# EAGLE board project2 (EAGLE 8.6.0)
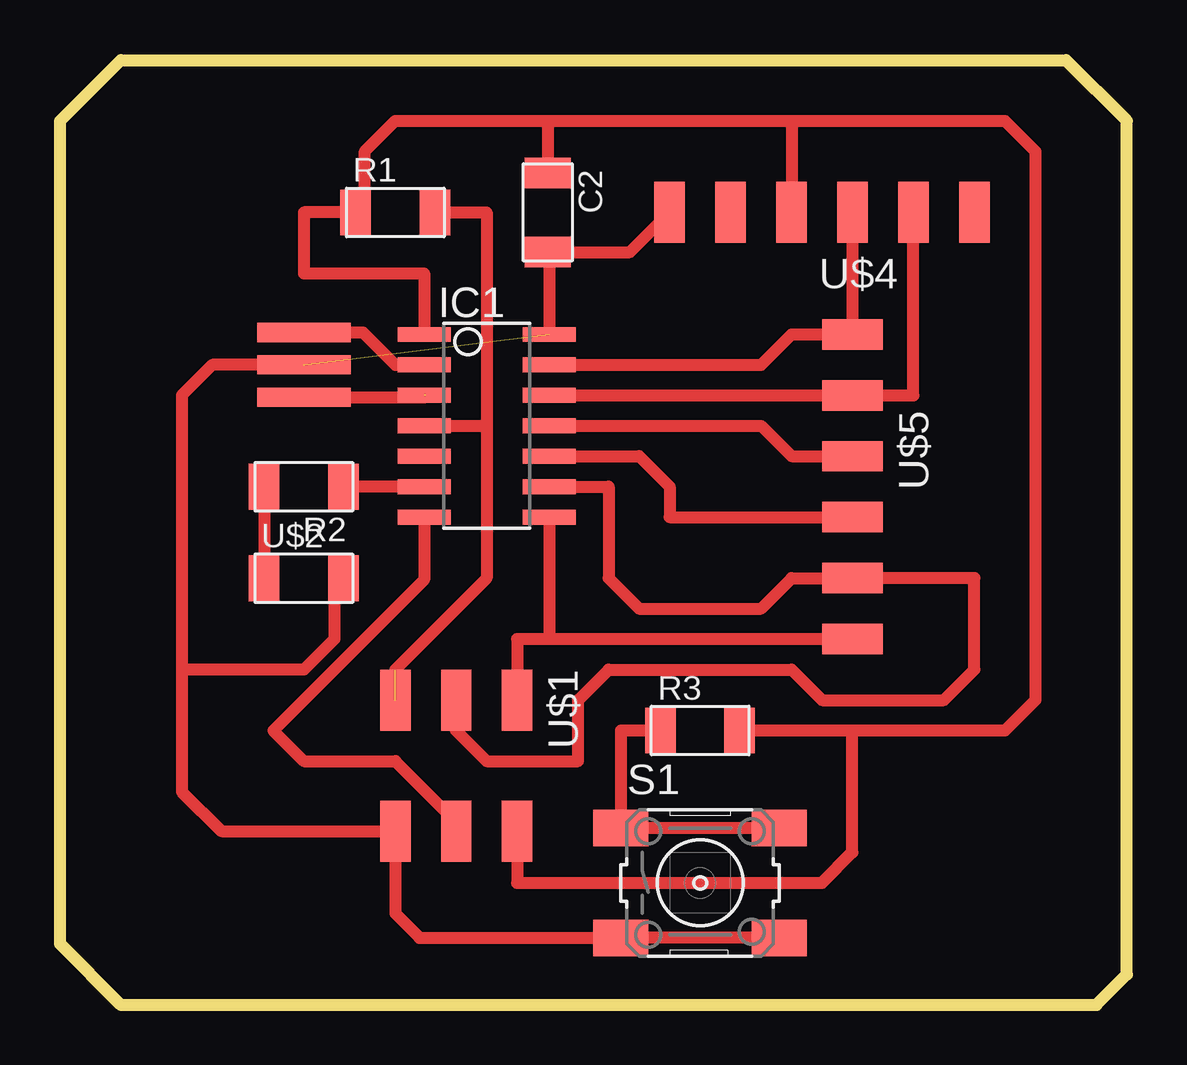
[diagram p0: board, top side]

Size 44.45 x 39.37 mm. Coordinates in mm from the lower left corner, seen from the top.
Outline: 2.54,0 43.18,0 44.45,1.27 44.45,36.83 41.91,39.37 2.54,39.37 0,36.83 0,2.54 2.54,0
Copper layers (1*16): Top 0.035mm / dielectric 1.5mm / Bottom 0.035mm
Design rules "default": minimum track width 6mil, minimum drill 0.35mm, track to track 6mil, track to pad 6mil, pad to pad 6mil, via to via 6mil, smd to smd 6mil, copper to edge 40mil, drill to drill 6mil, minimum pad ring 10mil, minimum via ring 8mil, stop-mask expansion 4mil, vias tented up to drill 0mil, thermal gap 10mil

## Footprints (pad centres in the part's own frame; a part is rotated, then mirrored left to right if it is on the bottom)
C1206FAB = smd 1.27 x 1.905: 1 -1.651,0; 2 1.651,0
SOIC14 = smd 0.61 x 2.21: 1 -3.81,-2.603; 2 -2.54,-2.603; 3 -1.27,-2.603; 4 0,-2.603; 5 1.27,-2.603; 6 2.54,-2.603; 7 3.81,-2.603; 8 3.81,2.603; 9 2.54,2.603; 10 1.27,2.603; 11 0,2.603; 12 -1.27,2.603; 13 -2.54,2.603; 14 -3.81,2.603
R1206FAB = smd 1.27 x 1.905: 1 -1.651,0; 2 1.651,0
6MM_SWITCH = smd 2.286 x 1.524: 1 -3.302,2.286; 2 3.302,2.286; 3 -3.302,-2.286; 4 3.302,-2.286
2X03SMD = smd 2.54 x 1.27: 1 -2.54,2.54; 2 2.92,2.54; 3 -2.54,0; 4 2.92,0; 5 -2.54,-2.54; 6 2.92,-2.54
LED1206FAB = smd 1.27 x 1.905: 1 -1.651,0; 2 1.651,0
EFOBM = smd 0.8 x 3.9: 1 -1.35,0; 2 0,0; 3 1.35,0
1X06SMD = smd 2.54 x 1.27: 1 0,6.35; 2 0,3.81; 3 0,1.27; 4 0,-1.27; 5 0,-3.81; 6 0,-6.35

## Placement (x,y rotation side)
C2  CAP-US1206FAB  [C1206FAB]  20.32,33.02 270 top
IC1  ATTINY44-SSU  [SOIC14]  17.78,24.13 270 top
R1  [R1206FAB]  13.97,33.02 0 top
R2  [R1206FAB]  10.16,21.59 180 top
R3  [R1206FAB]  26.67,11.43 0 top
S1  [6MM_SWITCH]  26.67,5.08 0 top
U$1  AVRISPSMD  [2X03SMD]  16.51,10.16 270 top
U$2  LEDFAB1206  [LED1206FAB]  10.16,17.78 0 top
U$3  RESONATOR  [EFOBM]  10.16,26.67 270 top
U$4  FTDI-SMD-HEADER  [1X06SMD]  31.75,33.02 90 top
U$5  FTDI-SMD-HEADER  [1X06SMD]  33.02,21.59 180 top

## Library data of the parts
C2 IC1 R1-R3 S1 U$1-U$5 = fab

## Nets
CTS: U$4.2
GND: C2.2 IC1.14 S1.3 S1.4 U$1.6 U$2.2 U$3.2 U$4.1
LED: IC1.6 R2.1
MISO: IC1.8 U$1.1 U$5.1
MOSI: IC1.7 U$1.4
N$1: R2.2 U$2.1
N$2: R3.1 S1.1 S1.2
N$3: IC1.3 U$3.3
N$4: IC1.2 U$3.1
N$7: IC1.10 U$5.3
N$8: IC1.11 U$5.4
RST: IC1.4 R1.2 U$1.5
RTS: U$4.6
RX: IC1.12 U$4.5 U$5.5
SCK: IC1.9 U$1.3 U$5.2
TX: IC1.13 U$4.4 U$5.6
VCC: C2.1 IC1.1 R1.1 R3.2 U$1.2 U$4.3

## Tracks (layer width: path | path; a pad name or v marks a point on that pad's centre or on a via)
GND  (1 unrouted)
  Top 0.508: S1.4 24.13,2.79 S1.3 14.99,2.79 13.97,3.81 U$1.6 6.73,7.24 5.08,8.89 5.08,13.97 | IC1.14 20.38,31.37 C2.2 23.75,31.37 U$4.1 | U$2.2 11.43,17.4 11.43,15.24 10.16,13.97 5.08,13.97 | U$3.2 6.35,26.67 5.08,25.4 5.08,13.97
LED
  Top 0.508: IC1.6 R2.1
MISO
  Top 0.508: IC1.8 20.38,15.24 | 20.38,15.24 19.05,15.24 U$1.1 | U$5.1 20.38,15.24
MOSI
  Top 0.508: IC1.7 15.18,17.72 8.89,11.43 10.16,10.16 13.97,10.16 16.51,7.62 U$1.4
N$1
  Top 0.508: R2.2 U$2.1 8.89,17.78
N$2
  Top 0.508: S1.2 S1.1 23.37,11.43 R3.1
N$3  (1 unrouted)
  Top 0.508: U$3.3 15.24,25.32 15.24,25.4
N$4
  Top 0.508: 10.16,27.94 U$3.1 12.62,28.02 13.97,26.67 IC1.2
N$7
  Top 0.508: IC1.10 24.13,22.86 25.4,21.59 25.4,20.32 U$5.3
N$8
  Top 0.508: IC1.11 29.21,24.13 30.48,22.86 U$5.4
RST  (1 unrouted)
  Top 0.508: 15.24,33.02 R1.2 17.78,33.02 17.78,24.13 | IC1.4 17.78,24.13 | 17.78,24.13 17.78,17.78 13.97,13.97
RX
  Top 0.508: IC1.12 U$5.5 35.56,25.4 U$4.5
SCK
  Top 0.508: U$1.3 16.51,11.43 17.78,10.16 21.59,10.16 21.59,12.7 22.86,13.97 30.48,13.97 31.75,12.7 36.83,12.7 38.1,13.97 38.1,17.78 U$5.2 30.48,17.78 29.21,16.51 24.13,16.51 22.86,17.78 22.86,21.59 IC1.9
TX
  Top 0.508: U$4.4 U$5.6 30.48,27.94 29.21,26.67 IC1.13
VCC
  Top 0.508: R1.1 12.7,33.02 | 20.32,36.83 C2.1 | 20.32,36.83 30.48,36.83 | 30.48,36.83 U$4.3 | U$1.2 19.05,5.08 31.75,5.08 33.02,6.35 33.02,11.43 | R1.1 10.16,33.02 10.16,30.48 15.18,30.48 IC1.1 | R1.1 12.7,33.4 12.7,35.56 13.97,36.83 20.32,36.83 | 30.48,36.83 39.37,36.83 40.64,35.56 40.64,34.29 40.64,33.02 40.64,12.7 39.37,11.43 33.02,11.43 | 33.02,11.43 R3.2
